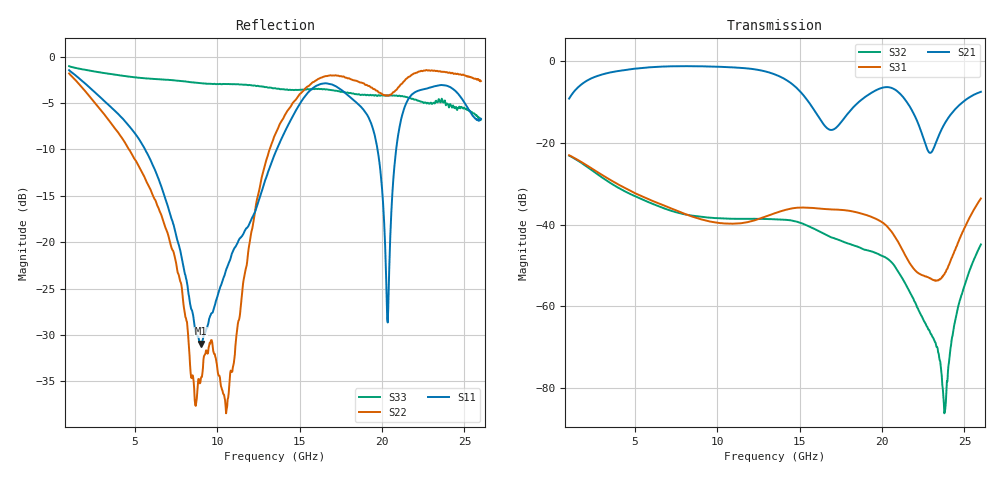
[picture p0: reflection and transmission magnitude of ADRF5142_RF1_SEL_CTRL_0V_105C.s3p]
! Device: ADRF5142
! Description: Silicon, SPDT Switch, Reflective
! Frequency: 8.00 GHz - 11.00 GHz
! Ports:
!  RFC = Port 1
!  RF1 = Port 2
!  RF2 = Port 3
! VDD = +3.3V
! VSS = -3.3V
! CTRL = 0V
! Temp = 105C
! Data:  Data was collected using an calibrated 4 port network analyzer.
!  The reference plane is the package pins of ADRF5142 switch.
! Notes: Analog Devices supplies this data as a sample of measured data
!  for this product.  Your particular data for this product may vary.
!  Data was taken at 105 degrees C.
!  Analog Devices reserves the right to change this data at anytime.
# HZ S DB R 50
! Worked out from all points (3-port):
!   801 points, 1 GHz to 26 GHz, reference 50 ohm
!   strongest paths, dB at 1 GHz, 7.25 GHz, 13.5 GHz, 19.75 GHz, 26 GHz:
!     S21: -9.1, -1.2, -3.2, -6.9, -7.5
!     S31: -23.0, -36.1, -37.2, -38.8, -33.6
!     S32: -23.1, -36.7, -38.7, -47.2, -44.9
!   lowest |S11| = -30.9 dB at 9 GHz (marker M1), VSWR 1.06, Z = 48.7 + j2.48 ohm
!   |S11| at or under -10 dB: 5.614 GHz to 13.6 GHz (7.991 GHz wide, 83.2 % of centre); 19.73 GHz to 20.86 GHz (1.131 GHz wide, 5.57 % of centre)
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1e9  -1.45 158.2  -9.13 35.5  -23.01 -37.0
     -9.13 35.5  -1.81 125.2  -23.11 -54.6
     -23.01 -37.0  -23.11 -54.6  -1.02 170.6
3.0937e9  -4.70 126.5  -3.12 -22.1  -28.05 -89.2
          -3.12 -22.1  -6.12 30.6  -28.71 -143.2
          -28.05 -89.2  -28.71 -143.2  -1.75 155.7
9e9  -30.94 116.3  -1.22 -157.2  -38.68 -154.9
     -1.22 -157.2  -34.67 122.0  -38.07 64.3
     -38.68 -154.9  -38.07 64.3  -2.86 121.0
1.35e10  -10.43 -120.1  -3.22 90.6  -37.19 177.6
         -3.22 90.6  -8.42 67.0  -38.67 -46.8
         -37.19 177.6  -38.67 -46.8  -3.39 91.7
1.6375e10  -2.90 168.1  -15.02 38.6  -36.14 121.0
           -15.02 38.6  -2.22 -30.0  -42.05 -142.9
           -36.14 121.0  -42.05 -142.9  -3.52 69.0
1.88437e10  -5.64 92.3  -9.13 62.6  -37.41 71.3
            -9.13 62.6  -2.85 -88.4  -46.01 138.9
            -37.41 71.3  -46.01 138.9  -4.10 50.0
2.03437e10  -28.64 135.4  -6.32 11.3  -40.59 34.3
            -6.32 11.3  -4.17 -106.7  -48.39 78.3
            -40.59 34.3  -48.39 78.3  -4.18 36.5
2.18125e10  -4.07 153.4  -11.99 -46.6  -50.23 31.9
            -11.99 -46.6  -1.95 -122.0  -57.51 21.4
            -50.23 31.9  -57.51 21.4  -4.55 26.8
2.37812e10  -3.08 63.4  -15.39 19.0  -52.20 122.3
            -15.39 19.0  -1.63 -163.5  -86.22 -63.6
            -52.20 122.3  -86.22 -63.6  -4.85 0.9
2.6e10  -6.68 -38.9  -7.46 -30.8  -33.59 128.1
        -7.46 -30.8  -2.63 160.8  -44.86 134.8
        -33.59 128.1  -44.86 134.8  -6.78 -12.8
